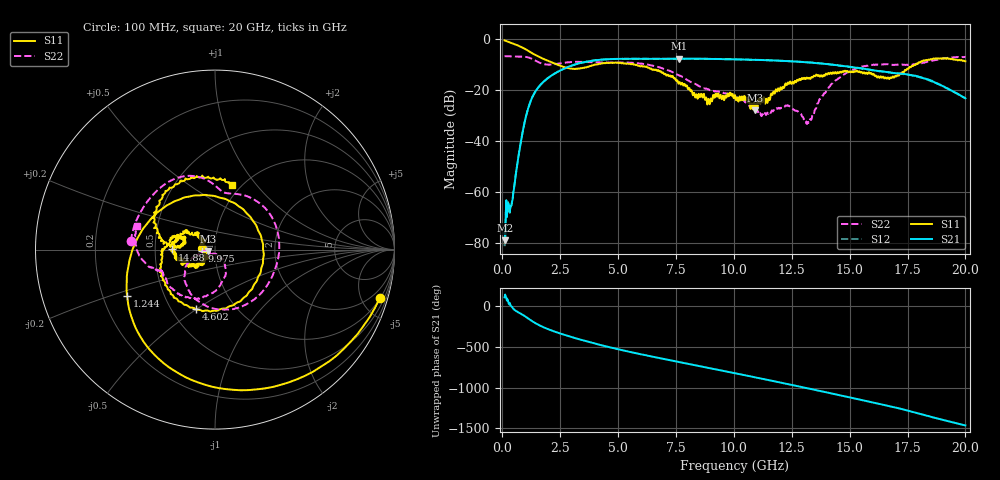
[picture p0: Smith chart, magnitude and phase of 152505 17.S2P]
!  2-Port S-parameters saved by WinCal
! VAR MeasName=S-Parameters (CALIBRATED_DATA) read from VNA (N5230C)
! VAR MeasDate=4/10/2015 9:30:01 AM
! VAR NAME=152505 17
! VAR FILENAME=152505 17.S2P
! VAR DATE=4/10/2015 9:30:01 AM
! VAR PHYS_PORTS=1,2
# Hz S DB R 50
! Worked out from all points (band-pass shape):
!   801 points, 100 MHz to 20 GHz, reference 50 ohm
!   highest |S21| = -7.51 dB at 7.637 GHz (marker M1); lowest = -78.7 dB at 124.9 MHz (marker M2)
!   |S21| within 3 dB of the highest: 2.918 GHz to 14.8 GHz (11.88 GHz wide, 134 % of centre)
!   lowest |S11| = -27.8 dB at 10.92 GHz (marker M3), VSWR 1.08, Z = 46.2 - j0.871 ohm
!   |S11| at or under -10 dB: 2.413 GHz to 3.956 GHz (1.543 GHz wide, 48.5 % of centre); 5.746 GHz to 5.79 GHz (43.94 MHz wide, 0.762 % of centre); 5.809 GHz to 17.78 GHz (11.97 GHz wide, 101 % of centre)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
!   |S22| runs from -33.1 to -6.5 dB; largest |S21 - S12| = 0.0075
!   S11 on the Smith chart (normalised r, x): 100 MHz: 1.05, -6.80; 1.244 GHz: 0.30, -0.22; 4.602 GHz: 0.66, -0.50; 9.975 GHz: 0.86, -0.01; 14.88 GHz: 0.61, +0.00; 20 GHz: 0.91, +0.76
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1e8  -0.38 -16.4  -75.87 107.5  -81.10 82.9  -6.55 174.3
1.24875e8  -0.46 -20.0  -78.73 142.1  -74.19 103.5  -6.55 172.8
4.23375e8  -1.44 -60.7  -63.57 -10.7  -63.38 -15.3  -6.64 155.8
5.975e8  -2.07 -82.4  -52.07 -61.6  -52.09 -60.8  -6.70 146.0
9.20875e8  -3.40 -119.9  -34.36 -113.5  -34.31 -113.4  -6.76 126.9
1.24425e9  -5.15 -152.4  -23.74 -176.0  -23.70 -176.1  -7.44 105.4
2.363625e9  -9.78 111.9  -12.83 37.7  -12.81 37.4  -9.54 68.1
3.43325e9  -11.29 -10.8  -9.09 -55.5  -9.11 -55.4  -8.78 20.8
4.602375e9  -9.13 -107.8  -7.72 -142.2  -7.74 -142.3  -9.08 -27.1
5.52275e9  -9.54 -153.8  -7.58 158.2  -7.57 158.1  -9.10 -64.2
6.741625e9  -12.05 162.9  -7.58 85.8  -7.56 85.4  -10.79 -115.7
7.637125e9  -17.00 138.8  -7.51 34.1  -7.55 34.4  -14.06 -146.8
8.880875e9  -24.49 161.3  -7.59 -36.7  -7.59 -36.5  -19.53 -162.3
9.975375e9  -22.51 -176.0  -7.75 -99.0  -7.80 -99.0  -22.17 -170.0
1.005e10  -21.83 -179.8  -7.78 -103.3  -7.80 -103.4  -22.43 -171.4
1.092062e10  -27.81 -166.6  -8.00 -153.1  -8.00 -152.9  -27.16 -170.4
1.231362e10  -17.17 -140.2  -8.47 125.4  -8.43 124.9  -25.87 -133.9
1.338325e10  -14.84 -155.7  -9.12 60.7  -9.06 60.7  -29.99 -71.0
1.487575e10  -12.39 179.9  -10.57 -31.1  -10.56 -31.5  -13.07 -86.9
1.669162e10  -15.39 169.2  -12.85 -145.2  -12.92 -145.9  -9.76 -144.6
1.83085e10  -8.00 148.8  -15.56 99.3  -15.40 98.0  -8.90 -163.5
2e10  -8.55 75.3  -23.08 -23.3  -23.12 -22.4  -6.88 162.8
